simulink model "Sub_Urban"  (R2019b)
settings: Solver=FixedStepAuto  StartTime=0.0  StopTime=3600*24  FixedStep=Tstep  MaxStep=1800  RelTol=1e-3
InitFcn:
  | load('network_parameters')
  | Vnom=400/sqrt(3);
  | Tstep=30*60;
  | MV_LV_transf=0;
StopFcn:
  | run('Simulink_Data.m')
undefined symbols (not defined in the file or in its folder): C_xlpe_185_90, D11, Delta, L_2x16mm, L_2x22mm, L_4x100mm, L_4x16mm, L_4x22mm, L_4x50mm, L_xlpe_185_90, LC, Line_length, R_2x16mm, R_2x22mm, R_4x100mm, R_4x16mm, R_4x22mm, R_4x50mm, R_xlpe_185_90, Source_Voltage
libraries: myLibrary x125, powerlib x89
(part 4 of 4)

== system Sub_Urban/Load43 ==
  SPDL - Single Phase Dynamic Load (Phasor) : myLibrary/SPDL - Single Phase Dynamic Load (Phasor)  Load_Profile=LC(43)  Phase=1
  Ph : PMIOPort  Side=Left
  n : PMIOPort  Port=2  Side=Left
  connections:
  Ph/RConn1 -- SPDL - Single Phase Dynamic Load (Phasor)/LConn1
  n/RConn1 -- SPDL - Single Phase Dynamic Load (Phasor)/LConn2

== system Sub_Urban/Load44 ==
  SPDL - Single Phase Dynamic Load (Phasor) : myLibrary/SPDL - Single Phase Dynamic Load (Phasor)  Load_Profile=LC(44)  Phase=3
  Ph : PMIOPort  Side=Left
  n : PMIOPort  Port=2  Side=Left
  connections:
  Ph/RConn1 -- SPDL - Single Phase Dynamic Load (Phasor)/LConn1
  n/RConn1 -- SPDL - Single Phase Dynamic Load (Phasor)/LConn2

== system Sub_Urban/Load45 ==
  SPDL - Single Phase Dynamic Load (Phasor) : myLibrary/SPDL - Single Phase Dynamic Load (Phasor)  Load_Profile=LC(45)  Phase=2
  Ph : PMIOPort  Side=Left
  n : PMIOPort  Port=2  Side=Left
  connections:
  Ph/RConn1 -- SPDL - Single Phase Dynamic Load (Phasor)/LConn1
  n/RConn1 -- SPDL - Single Phase Dynamic Load (Phasor)/LConn2

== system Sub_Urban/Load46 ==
  SPDL - Single Phase Dynamic Load (Phasor) : myLibrary/SPDL - Single Phase Dynamic Load (Phasor)  Load_Profile=LC(46)  Phase=1
  Ph : PMIOPort  Side=Left
  n : PMIOPort  Port=2  Side=Left
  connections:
  Ph/RConn1 -- SPDL - Single Phase Dynamic Load (Phasor)/LConn1
  n/RConn1 -- SPDL - Single Phase Dynamic Load (Phasor)/LConn2

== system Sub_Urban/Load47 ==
  SPDL - Single Phase Dynamic Load (Phasor) : myLibrary/SPDL - Single Phase Dynamic Load (Phasor)  Load_Profile=LC(47)  Phase=2
  Ph : PMIOPort  Side=Left
  n : PMIOPort  Port=2  Side=Left
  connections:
  Ph/RConn1 -- SPDL - Single Phase Dynamic Load (Phasor)/LConn1
  n/RConn1 -- SPDL - Single Phase Dynamic Load (Phasor)/LConn2

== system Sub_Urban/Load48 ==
  SPDL - Single Phase Dynamic Load (Phasor) : myLibrary/SPDL - Single Phase Dynamic Load (Phasor)  Load_Profile=LC(48)  Phase=3
  Ph : PMIOPort  Side=Left
  n : PMIOPort  Port=2  Side=Left
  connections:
  Ph/RConn1 -- SPDL - Single Phase Dynamic Load (Phasor)/LConn1
  n/RConn1 -- SPDL - Single Phase Dynamic Load (Phasor)/LConn2

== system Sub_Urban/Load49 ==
  TPDL - Three-Phase Dynamic Load : myLibrary/TPDL - Three-Phase Dynamic Load  Load_Profile=LC(49)
  A : PMIOPort  Side=Left
  B : PMIOPort  Port=2  Side=Left
  C : PMIOPort  Port=3  Side=Left
  n : PMIOPort  Port=4  Side=Left
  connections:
  A/RConn1 -- TPDL - Three-Phase Dynamic Load/LConn1
  TPDL - Three-Phase Dynamic Load/LConn2 -- B/RConn1
  C/RConn1 -- TPDL - Three-Phase Dynamic Load/LConn3
  n/RConn1 -- TPDL - Three-Phase Dynamic Load/LConn4

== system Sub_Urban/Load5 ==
  SPDL - Single Phase Dynamic Load (Phasor) : myLibrary/SPDL - Single Phase Dynamic Load (Phasor)  Load_Profile=LC(5)  Phase=3
  Ph : PMIOPort  Side=Left
  n : PMIOPort  Port=2  Side=Left
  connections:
  Ph/RConn1 -- SPDL - Single Phase Dynamic Load (Phasor)/LConn1
  n/RConn1 -- SPDL - Single Phase Dynamic Load (Phasor)/LConn2

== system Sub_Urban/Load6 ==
  SPDL - Single Phase Dynamic Load (Phasor) : myLibrary/SPDL - Single Phase Dynamic Load (Phasor)  Load_Profile=LC(6)  Phase=2
  Ph : PMIOPort  Side=Left
  n : PMIOPort  Port=2  Side=Left
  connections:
  Ph/RConn1 -- SPDL - Single Phase Dynamic Load (Phasor)/LConn1
  n/RConn1 -- SPDL - Single Phase Dynamic Load (Phasor)/LConn2

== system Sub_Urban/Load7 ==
  SPDL - Single Phase Dynamic Load (Phasor) : myLibrary/SPDL - Single Phase Dynamic Load (Phasor)  Load_Profile=LC(7)  Phase=2
  Ph : PMIOPort  Side=Left
  n : PMIOPort  Port=2  Side=Left
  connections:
  Ph/RConn1 -- SPDL - Single Phase Dynamic Load (Phasor)/LConn1
  n/RConn1 -- SPDL - Single Phase Dynamic Load (Phasor)/LConn2

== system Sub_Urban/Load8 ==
  SPDL - Single Phase Dynamic Load (Phasor) : myLibrary/SPDL - Single Phase Dynamic Load (Phasor)  Load_Profile=LC(8)  Phase=1
  Ph : PMIOPort  Side=Left
  n : PMIOPort  Port=2  Side=Left
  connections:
  Ph/RConn1 -- SPDL - Single Phase Dynamic Load (Phasor)/LConn1
  n/RConn1 -- SPDL - Single Phase Dynamic Load (Phasor)/LConn2

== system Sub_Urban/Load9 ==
  SPDL - Single Phase Dynamic Load (Phasor) : myLibrary/SPDL - Single Phase Dynamic Load (Phasor)  Load_Profile=LC(9)  Phase=1
  Ph : PMIOPort  Side=Left
  n : PMIOPort  Port=2  Side=Left
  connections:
  Ph/RConn1 -- SPDL - Single Phase Dynamic Load (Phasor)/LConn1
  n/RConn1 -- SPDL - Single Phase Dynamic Load (Phasor)/LConn2

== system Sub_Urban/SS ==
  Ground1 : powerlib/Elements/Ground  LConnTagsString=a
  Normal : Subsystem
  OLTC : Subsystem  Commented=on
  Three-Phase Programmable Voltage Source : powerlib/Electrical Sources/Three-Phase Programmable Voltage Source  PositiveSequence=[11e3 0 50]  VariationEntity=None  VariationType=Table of time-amplitude pairs  VariationTypeAlt=Step  VariationStep=0.5  VariationRate=10  VariationMagnitude=0.3  VariationFrequency=2  VariationTiming=[1 2]  VariationPhaseA=off  Amplitudes=[1]  TimeValues=[0]  HarmonicGeneration=off  HarmonicA=[5 0.05 -25 2]  HarmonicB=[7 0.04 0 1]  Timing="[10  20]"  BusType=swing  Pref=0  Qref=0  Qmin=-inf  Qmax=inf
  A : PMIOPort  Tag=PMCPort  Side=Right
  B : PMIOPort  Tag=PMCPort  Port=2  Side=Right
  C : PMIOPort  Tag=PMCPort  Port=3  Side=Right
  N : PMIOPort  Tag=PMCPort  Port=4  Side=Right
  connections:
  Three-Phase Programmable Voltage Source/LConn1 -- Normal/RConn4 -- N/RConn1 -- OLTC/RConn4 -- Ground1/LConn1
  A/RConn1 -- OLTC/RConn1 -- Normal/RConn1
  B/RConn1 -- Normal/RConn2 -- OLTC/RConn2
  C/RConn1 -- Normal/RConn3 -- OLTC/RConn3

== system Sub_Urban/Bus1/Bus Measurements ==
  Vabcn : Inport
  Iabc : Inport  Port=2
  Complex to Magnitude-Angle : ComplexToMagnitudeAngle
  Complex to Magnitude-Angle1 : ComplexToMagnitudeAngle
  Mux : Mux  Inputs=2
  Mux1 : Mux  Inputs=2
  Rad->Deg.2 : Gain  Gain=180/pi
  Rad->Deg.3 : Gain  Gain=180/pi
  To Workspace : ToWorkspace  VariableName=Bus1  SaveFormat=Structure With Time  SampleTime=-1
  To Workspace1 : ToWorkspace  VariableName=I1  SaveFormat=Structure With Time  SampleTime=-1
  to RMS : Gain  Gain=1/sqrt(2)
  to RMS.2 : Gain  Gain=1/sqrt(2)
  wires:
  Complex to Magnitude-Angle/1 -> to RMS/1
  Mux/1 -> To Workspace/1
  Mux1/1 -> To Workspace1/1
  to RMS/1 -> Mux/1
  Rad->Deg.2/1 -> Mux/2
  Vabcn/1 -> Complex to Magnitude-Angle/1
  Complex to Magnitude-Angle/2 -> Rad->Deg.2/1
  Iabc/1 -> Complex to Magnitude-Angle1/1
  Complex to Magnitude-Angle1/1 -> to RMS.2/1
  Complex to Magnitude-Angle1/2 -> Rad->Deg.3/1
  Rad->Deg.3/1 -> Mux1/2
  to RMS.2/1 -> Mux1/1

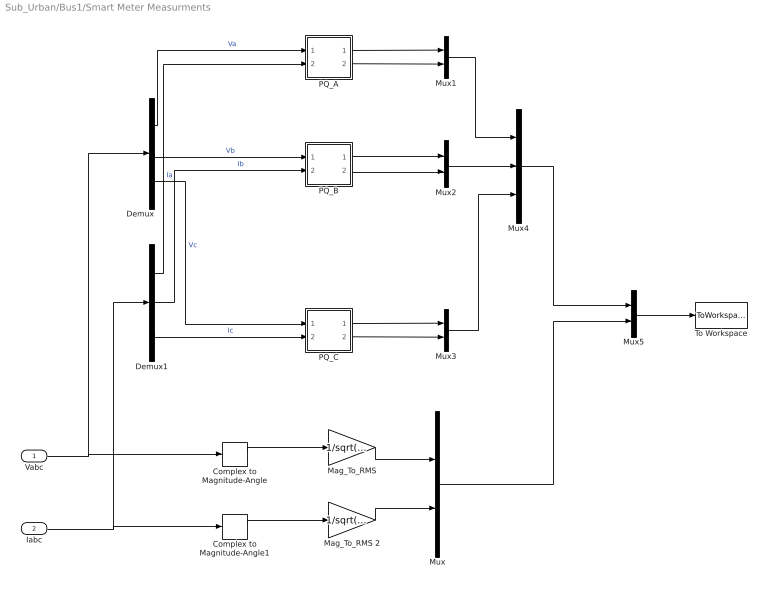
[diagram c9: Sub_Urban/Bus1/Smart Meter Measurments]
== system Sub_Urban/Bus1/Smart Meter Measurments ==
  Vabc : Inport
  Iabc : Inport  Port=2
  Complex to Magnitude-Angle : ComplexToMagnitudeAngle
  Complex to Magnitude-Angle1 : ComplexToMagnitudeAngle
  Demux : Demux  Outputs=3
  Demux1 : Demux  Outputs=3
  Mag_To_RMS : Gain  Gain=1/sqrt(2)
  Mag_To_RMS 2 : Gain  Gain=1/sqrt(2)
  Mux{,1..3,5} (5 alike) : Mux  Inputs=2
  Mux4 : Mux  Inputs=3
  PQ_A : Subsystem
  PQ_B : Subsystem
  PQ_C : Subsystem
  To Workspace : ToWorkspace  VariableName=Bus1gen  SaveFormat=Structure With Time  SampleTime=-1
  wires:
  PQ_A/1(P) -> Mux1/1
  PQ_A/2(Q) -> Mux1/2
  PQ_B/1(P) -> Mux2/1
  PQ_B/2(Q) -> Mux2/2
  PQ_C/1(P) -> Mux3/1
  PQ_C/2(Q) -> Mux3/2
  Mux1/1 -> Mux4/1
  Mux2/1 -> Mux4/2
  Mux5/1 -> To Workspace/1
  Mux/1 -> Mux5/2
  Mux3/1 -> Mux4/3
  Mux4/1 -> Mux5/1
  Vabc/1 -> Complex to Magnitude-Angle/1, Demux/1
  Iabc/1 -> Complex to Magnitude-Angle1/1, Demux1/1
  Complex to Magnitude-Angle/1 -> Mag_To_RMS/1
  Complex to Magnitude-Angle1/1 -> Mag_To_RMS 2/1
  Mag_To_RMS/1 -> Mux/1
  Mag_To_RMS 2/1 -> Mux/2
  Demux/1 -> PQ_A/1(V)  "Va"
  Demux1/1 -> PQ_A/2(I)  "Ia"
  Demux/2 -> PQ_B/1(V)  "Vb"
  Demux1/2 -> PQ_B/2(I)  "Ib"
  Demux/3 -> PQ_C/1(V)  "Vc"
  Demux1/3 -> PQ_C/2(I)  "Ic"

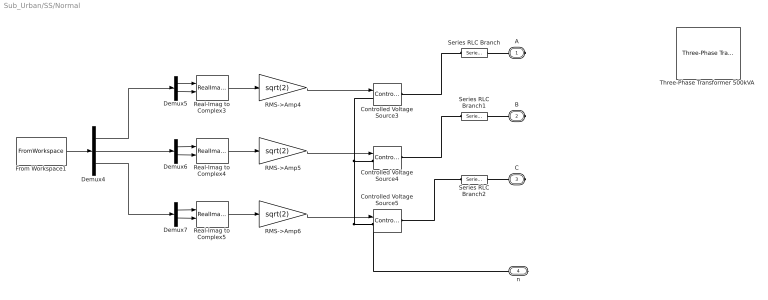
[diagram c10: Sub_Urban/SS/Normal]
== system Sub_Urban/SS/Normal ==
  Controlled Voltage Source3 : powerlib/Electrical Sources/Controlled Voltage Source  Initialize=off  Source_Type=AC  Amplitude=10  Phase=0  Frequency=50  Measurements=None
  Controlled Voltage Source4 : powerlib/Electrical Sources/Controlled Voltage Source  Initialize=off  Source_Type=AC  Amplitude=10  Phase=0  Frequency=50  Measurements=None
  Controlled Voltage Source5 : powerlib/Electrical Sources/Controlled Voltage Source  Initialize=off  Source_Type=AC  Amplitude=10  Phase=0  Frequency=50  Measurements=None
  Demux4 : Demux  Outputs=3
  Demux5 : Demux  Outputs=2
  Demux6 : Demux  Outputs=2
  Demux7 : Demux  Outputs=2
  From Workspace1 : FromWorkspace  VariableName=Source_Voltage  SampleTime=0  OutputAfterFinalValue=Holding final value
  RMS->Amp4 : Gain  Gain=sqrt(2)
  RMS->Amp5 : Gain  Gain=sqrt(2)
  RMS->Amp6 : Gain  Gain=sqrt(2)
  Real-Imag to Complex3 : RealImagToComplex
  Real-Imag to Complex4 : RealImagToComplex
  Real-Imag to Complex5 : RealImagToComplex
  Series RLC Branch : powerlib/Elements/Series RLC Branch  LConnTagsString=__new0  RConnTagsString=__new0  BranchType=R  Resistance=1e-4  Inductance=1e-3  SetiL0=off  InitialCurrent=0  Capacitance=1e-6  Setx0=off  InitialVoltage=0  Measurements=None
  Series RLC Branch1 : powerlib/Elements/Series RLC Branch  LConnTagsString=__new0  RConnTagsString=__new0  BranchType=R  Resistance=1e-4  Inductance=1e-3  SetiL0=off  InitialCurrent=0  Capacitance=1e-6  Setx0=off  InitialVoltage=0  Measurements=None
  Series RLC Branch2 : powerlib/Elements/Series RLC Branch  LConnTagsString=__new0  RConnTagsString=__new0  BranchType=R  Resistance=1e-4  Inductance=1e-3  SetiL0=off  InitialCurrent=0  Capacitance=1e-6  Setx0=off  InitialVoltage=0  Measurements=None
  "Three-Phase Transformer 500kVA " : powerlib/Elements/Three-Phase Transformer (Two Windings)  Commented=on  Winding1Connection=Delta (D11)  Winding2Connection=Yn  CoreType=Three single-phase transformers  SetSaturation=off  Hysteresis=off  DataFile='hysteresis'  SetInitialFlux=off  Measurements=None  UNITS=pu  NominalPower=[500e3 , 50]  Winding1=[11e3, 0.0092, 0.04660054]  Winding2=[Vnom*sqrt(3), 0.0092, 0.04660054]  Rm=499.99  Lm=500  L0=5.7388  Saturation=[0 0;0.00046184 6.235;0.19245 7.898]  InitialFluxes=[4.1569 -4.1569 3.6373]  BreakLoop=off  DiscreteSolver=Trapezoidal iterative  DataType=off  TransfoNumber=1
  A : PMIOPort  Tag=PMCPort  Side=Right
  B : PMIOPort  Tag=PMCPort  Port=2  Side=Right
  C : PMIOPort  Tag=PMCPort  Port=3  Side=Right
  n : PMIOPort  Port=4  Side=Right
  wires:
  Demux7/2 -> Real-Imag to Complex5/2
  RMS->Amp4/1 -> Controlled Voltage Source3/1
  Demux5/2 -> Real-Imag to Complex3/2
  Demux6/2 -> Real-Imag to Complex4/2
  Real-Imag to Complex5/1 -> RMS->Amp6/1
  Demux7/1 -> Real-Imag to Complex5/1
  Demux4/2 -> Demux6/1
  Demux5/1 -> Real-Imag to Complex3/1
  Demux6/1 -> Real-Imag to Complex4/1
  RMS->Amp5/1 -> Controlled Voltage Source4/1
  Real-Imag to Complex3/1 -> RMS->Amp4/1
  RMS->Amp6/1 -> Controlled Voltage Source5/1
  Real-Imag to Complex4/1 -> RMS->Amp5/1
  Demux4/1 -> Demux5/1
  From Workspace1/1 -> Demux4/1
  Demux4/3 -> Demux7/1
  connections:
  Controlled Voltage Source4/LConn1 -- Controlled Voltage Source3/LConn1 -- n/RConn1 -- Controlled Voltage Source5/LConn1
  B/RConn1 -- Series RLC Branch1/RConn1
  Series RLC Branch/RConn1 -- A/RConn1
  C/RConn1 -- Series RLC Branch2/RConn1
  Series RLC Branch/LConn1 -- Controlled Voltage Source3/RConn1
  Series RLC Branch1/LConn1 -- Controlled Voltage Source4/RConn1
  Series RLC Branch2/LConn1 -- Controlled Voltage Source5/RConn1

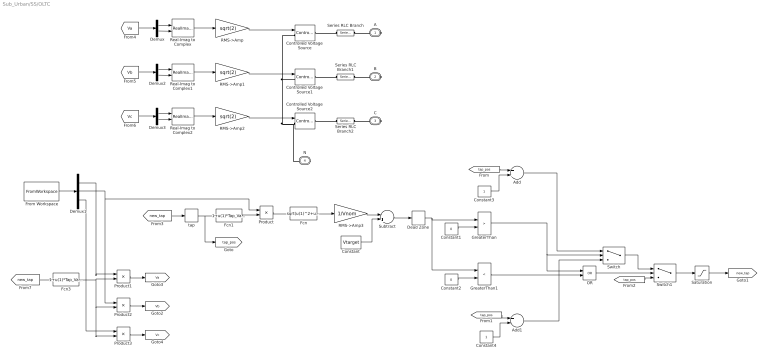
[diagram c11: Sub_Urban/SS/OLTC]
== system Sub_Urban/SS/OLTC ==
  Add : Sum
  Add1 : Sum  Inputs=+-
  Constant : Constant  Value=Vtarget
  Constant1 : Constant  Value=0
  Constant2 : Constant  Value=0
  Constant3 : Constant
  Constant4 : Constant
  Controlled Voltage Source : powerlib/Electrical Sources/Controlled Voltage Source  Initialize=off  Source_Type=AC  Amplitude=10  Phase=0  Frequency=50  Measurements=None
  Controlled Voltage Source1 : powerlib/Electrical Sources/Controlled Voltage Source  Initialize=off  Source_Type=AC  Amplitude=10  Phase=0  Frequency=50  Measurements=None
  Controlled Voltage Source2 : powerlib/Electrical Sources/Controlled Voltage Source  Initialize=off  Source_Type=AC  Amplitude=10  Phase=0  Frequency=50  Measurements=None
  Dead Zone : DeadZone  LowerValue=-deadband  UpperValue=deadband
  Demux : Demux  Outputs=2
  Demux1 : Demux  Outputs=3
  Demux2 : Demux  Outputs=2
  Demux3 : Demux  Outputs=2
  Fcn : Fcn  Expr=sqrt(u(1)^2+u(2)^2)
  Fcn1 : Fcn  Expr=1+u(1)*Tap_Value
  Fcn3 : Fcn  Expr=1+u(1)*Tap_Value
  From Workspace : FromWorkspace  VariableName=Source_Voltage  SampleTime=0  Interpolate=off  OutputAfterFinalValue=Holding final value
  GreaterThan : RelationalOperator  Operator=>  OutDataTypeStr=boolean  RndMeth=Simplest
  GreaterThan1 : RelationalOperator  Operator=<  OutDataTypeStr=boolean  RndMeth=Simplest
  OR : Logic  Operator=OR  IconShape=distinctive  AllPortsSameDT=off  OutDataTypeStr=boolean
  Product{,1..3} (4 alike) : Product
  RMS->Amp : Gain  Gain=sqrt(2)
  RMS->Amp1 : Gain  Gain=sqrt(2)
  RMS->Amp2 : Gain  Gain=sqrt(2)
  RMS->Amp3 : Gain  Gain=1/Vnom
  Real-Imag to Complex : RealImagToComplex
  Real-Imag to Complex1 : RealImagToComplex
  Real-Imag to Complex2 : RealImagToComplex
  Saturation : Saturate  UpperLimit=tap_num/2  LowerLimit=-tap_num/2
  Series RLC Branch : powerlib/Elements/Series RLC Branch  LConnTagsString=__new0  RConnTagsString=__new0  BranchType=R  Resistance=1e-4  Inductance=1e-3  SetiL0=off  InitialCurrent=0  Capacitance=1e-6  Setx0=off  InitialVoltage=0  Measurements=None
  Series RLC Branch1 : powerlib/Elements/Series RLC Branch  LConnTagsString=__new0  RConnTagsString=__new0  BranchType=R  Resistance=1e-4  Inductance=1e-3  SetiL0=off  InitialCurrent=0  Capacitance=1e-6  Setx0=off  InitialVoltage=0  Measurements=None
  Series RLC Branch2 : powerlib/Elements/Series RLC Branch  LConnTagsString=__new0  RConnTagsString=__new0  BranchType=R  Resistance=1e-4  Inductance=1e-3  SetiL0=off  InitialCurrent=0  Capacitance=1e-6  Setx0=off  InitialVoltage=0  Measurements=None
  Subtract : Sum  Inputs=-+
  Switch : Switch  Criteria=u2 > Threshold
  Switch1 : Switch  Criteria=u2 > Threshold
  tap : Memory
  A : PMIOPort  Tag=PMCPort  Side=Right
  B : PMIOPort  Tag=PMCPort  Port=2  Side=Right
  C : PMIOPort  Tag=PMCPort  Port=3  Side=Right
  N : PMIOPort  Tag=PMCPort  Port=4  Side=Right
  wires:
  GreaterThan/1 -> OR/1, Switch/2
  Product/1 -> Fcn/1
  [tap_pos] -> Switch1/3
  Real-Imag to Complex2/1 -> RMS->Amp2/1
  Add1/1 -> Switch/3
  Demux1/2 -> Product2/1, Product/1
  Fcn3/1 -> Product3/2, Product2/2, Product1/2
  Saturation/1 -> [new_tap]
  Demux2/2 -> Real-Imag to Complex1/2
  [Vc] -> Demux3/1
  Switch/1 -> Switch1/1
  [tap_pos] -> Add/1
  Product2/1 -> [Vb]
  Fcn/1 -> RMS->Amp3/1
  Dead Zone/1 -> GreaterThan/1, GreaterThan1/1
  [Va] -> Demux/1
  Demux1/3 -> Product3/1
  RMS->Amp3/1 -> Subtract/1
  Real-Imag to Complex/1 -> RMS->Amp/1
  OR/1 -> Switch1/2
  Constant/1 -> Subtract/2
  GreaterThan1/1 -> OR/2
  RMS->Amp1/1 -> Controlled Voltage Source1/1
  Constant4/1 -> Add1/2
  Real-Imag to Complex1/1 -> RMS->Amp1/1
  RMS->Amp2/1 -> Controlled Voltage Source2/1
  Product3/1 -> [Vc]
  From Workspace/1 -> Demux1/1
  Subtract/1 -> Dead Zone/1
  tap/1 -> Fcn1/1, [tap_pos]
  Fcn1/1 -> Product/2
  Constant2/1 -> GreaterThan1/2
  [new_tap] -> Fcn3/1
  [tap_pos] -> Add1/1
  Constant3/1 -> Add/2
  Add/1 -> Switch/1
  Demux2/1 -> Real-Imag to Complex1/1
  Demux/1 -> Real-Imag to Complex/1
  Demux3/1 -> Real-Imag to Complex2/1
  Demux3/2 -> Real-Imag to Complex2/2
  Demux1/1 -> Product1/1
  [new_tap] -> tap/1
  Switch1/1 -> Saturation/1
  [Vb] -> Demux2/1
  Product1/1 -> [Va]
  Constant1/1 -> GreaterThan/2
  Demux/2 -> Real-Imag to Complex/2
  RMS->Amp/1 -> Controlled Voltage Source/1
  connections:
  Controlled Voltage Source/LConn1 -- N/RConn1 -- Controlled Voltage Source2/LConn1 -- Controlled Voltage Source1/LConn1
  Series RLC Branch1/LConn1 -- Controlled Voltage Source1/RConn1
  Series RLC Branch/LConn1 -- Controlled Voltage Source/RConn1
  Series RLC Branch/RConn1 -- A/RConn1
  C/RConn1 -- Series RLC Branch2/RConn1
  Controlled Voltage Source2/RConn1 -- Series RLC Branch2/LConn1
  B/RConn1 -- Series RLC Branch1/RConn1

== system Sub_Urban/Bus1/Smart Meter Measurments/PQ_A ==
  V : Inport
  I : Inport  Port=2
  Complex to Real-Imag : ComplexToRealImag
  Constant : Constant  Value=2
  Divide : Product  Inputs=*/
  Math Function : Math  Operator=conj
  Product : Product
  P : Outport  VectorParamsAs1DForOutWhenUnconnected=off
  Q : Outport  Port=2  VectorParamsAs1DForOutWhenUnconnected=off
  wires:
  I/1 -> Math Function/1
  V/1 -> Product/1
  Math Function/1 -> Product/2
  Product/1 -> Divide/1
  Constant/1 -> Divide/2
  Divide/1 -> Complex to Real-Imag/1
  Complex to Real-Imag/1 -> P/1
  Complex to Real-Imag/2 -> Q/1

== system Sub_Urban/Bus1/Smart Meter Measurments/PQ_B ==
  V : Inport
  I : Inport  Port=2
  Complex to Real-Imag : ComplexToRealImag
  Constant : Constant  Value=2
  Divide : Product  Inputs=*/
  Math Function : Math  Operator=conj
  Product : Product
  P : Outport  VectorParamsAs1DForOutWhenUnconnected=off
  Q : Outport  Port=2  VectorParamsAs1DForOutWhenUnconnected=off
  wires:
  I/1 -> Math Function/1
  V/1 -> Product/1
  Math Function/1 -> Product/2
  Product/1 -> Divide/1
  Constant/1 -> Divide/2
  Divide/1 -> Complex to Real-Imag/1
  Complex to Real-Imag/1 -> P/1
  Complex to Real-Imag/2 -> Q/1

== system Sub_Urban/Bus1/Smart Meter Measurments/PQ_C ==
  V : Inport
  I : Inport  Port=2
  Complex to Real-Imag : ComplexToRealImag
  Constant : Constant  Value=2
  Divide : Product  Inputs=*/
  Math Function : Math  Operator=conj
  Product : Product
  P : Outport  VectorParamsAs1DForOutWhenUnconnected=off
  Q : Outport  Port=2  VectorParamsAs1DForOutWhenUnconnected=off
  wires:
  I/1 -> Math Function/1
  V/1 -> Product/1
  Math Function/1 -> Product/2
  Product/1 -> Divide/1
  Constant/1 -> Divide/2
  Divide/1 -> Complex to Real-Imag/1
  Complex to Real-Imag/1 -> P/1
  Complex to Real-Imag/2 -> Q/1
